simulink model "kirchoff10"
settings: Solver=ode23s  StartTime=0.0  StopTime=1  RelTol=1e-3
libraries: fl_lib x14, nesl_utility x7, powerlib x1

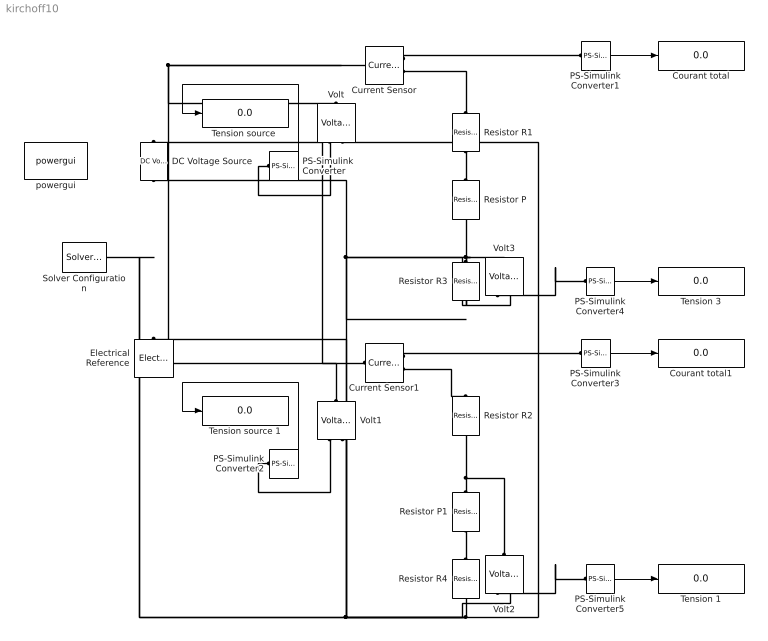
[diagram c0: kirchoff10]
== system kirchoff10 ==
  Courant total : Display
  Courant total1 : Display
  Current Sensor : fl_lib/Electrical/Electrical Sensors/Current Sensor  i1_Log=off  v1_Log=off  LocalVarNames=|i1|v1  LocalVarDescs=|i1|v1  LocalVarLogging=[0 0]
  Current Sensor1 : fl_lib/Electrical/Electrical Sensors/Current Sensor  i1_Log=off  v1_Log=off  LocalVarNames=|i1|v1  LocalVarDescs=|i1|v1  LocalVarLogging=[0 0]
  DC Voltage Source : fl_lib/Electrical/Electrical Sources/DC Voltage Source  v0=10 V  i_Log=off  v_Log=off  LocalVarNames=|i|v  LocalVarDescs=|i|v  LocalVarLogging=[0 0]
  Electrical Reference : fl_lib/Electrical/Electrical Elements/Electrical Reference  i_Log=off  LocalVarNames=|i  LocalVarDescs=|i  LocalVarLogging=0
  PS-Simulink Converter{,2,4..5} (4 alike) : nesl_utility/PS-Simulink Converter  PhysicalDomain=network_engine_domain  LeftPortType=input  RightPortType=output  SubClassName=ps_output  Unit=V  AffineConversion=off
  PS-Simulink Converter1 : nesl_utility/PS-Simulink Converter  PhysicalDomain=network_engine_domain  LeftPortType=input  RightPortType=output  SubClassName=ps_output  Unit=A  AffineConversion=off
  PS-Simulink Converter3 : nesl_utility/PS-Simulink Converter  PhysicalDomain=network_engine_domain  LeftPortType=input  RightPortType=output  SubClassName=ps_output  Unit=A  AffineConversion=off
  Resistor P : fl_lib/Electrical/Electrical Elements/Resistor  R=10 kOhm  i_Log=off  v_Log=off  LocalVarNames=|i|v  LocalVarDescs=|i|v  LocalVarLogging=[0 0]
  Resistor P1 : fl_lib/Electrical/Electrical Elements/Resistor  R=10 kOhm  i_Log=off  v_Log=off  LocalVarNames=|i|v  LocalVarDescs=|i|v  LocalVarLogging=[0 0]
  Resistor R{1..4} (4 alike) : fl_lib/Electrical/Electrical Elements/Resistor  R=100 Ohm  i_Log=off  v_Log=off  LocalVarNames=|i|v  LocalVarDescs=|i|v  LocalVarLogging=[0 0]
  Solver Configuration : nesl_utility/Solver Configuration  PhysicalDomain=network_engine_domain  LeftPortType=input  RightPortType=generic  SubClassName=solver  UseCustomDae=off  DoDC=off  ResidualTolerance=1e-9  UseLocalSolver=off  LocalSolverChoice=NE_BACKWARD_EULER_ADVANCER  LocalSolverSampleTime=.001  DoFixedCost=off  MaxNonlinIter=3  MaxModeIter=2  LinearAlgebra=Sparse  Accelerate=off  Profile=off  UseLocalSampling=off  DelaysMemoryBudget=1024
  Tension 1 : Display
  Tension 3 : Display
  "Tension source " : Display
  Tension source 1 : Display
  Volt{,1..3} (4 alike) : fl_lib/Electrical/Electrical Sensors/Voltage Sensor  i1_Log=off  v1_Log=off  LocalVarNames=|i1|v1  LocalVarDescs=|i1|v1  LocalVarLogging=[0 0]
  powergui : powerlib/powergui  Priority=1  SimulationMode=Continuous  SolverType=Tustin  SampleTime=50e-6  frequency=60  SPID=off  DisableSnubberDevices=off  DisableRonSwitches=off  DisableVfSwitches=off  SwTol=0  Interpol=off  DisplayEquations=off  FunctionMessages=off  frequencyindice=17  Pbase=100e6  ErrMax=1e-4  Iterations=50  UnitsV=V  UnitsW=W  echomessages=off  HookPort=off  EnableUseOfTLC=off  x0status=blocks  RestoreLinks=warning  ResistiveCurrentMeasurement=off  Ylog=off  Xlog=on  ShowGrid=off  save=off  variable=ZData  ZoomFFT=off  StartTime=0.0  cycles=1  DisplayStyle=1  FreqAxis=off  MaxFrequency=1000  frequencyindicesteady=1  display=off  methode=off
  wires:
  PS-Simulink Converter1/1 -> Courant total/1
  PS-Simulink Converter/1 -> "Tension source "/1
  PS-Simulink Converter4/1 -> Tension 3/1
  PS-Simulink Converter3/1 -> Courant total1/1
  PS-Simulink Converter2/1 -> Tension source 1/1
  PS-Simulink Converter5/1 -> Tension 1/1
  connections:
  Volt/LConn1 -- Current Sensor/LConn1 -- DC Voltage Source/LConn1 -- Current Sensor1/LConn1 -- Volt1/LConn1
  Current Sensor/RConn1 -- PS-Simulink Converter1/LConn1
  Resistor R1/LConn1 -- Current Sensor/RConn2
  Volt/RConn1 -- PS-Simulink Converter/LConn1
  Volt3/RConn1 -- PS-Simulink Converter4/LConn1
  Resistor R3/LConn1 -- Volt3/LConn1 -- Resistor P/RConn1
  Resistor R1/RConn1 -- Resistor P/LConn1
  Resistor R4/RConn1 -- Volt2/RConn2 -- Volt1/RConn2 -- Volt3/RConn2 -- Resistor R3/RConn1 -- Volt/RConn2 -- Solver Configuration/RConn1 -- DC Voltage Source/RConn1 -- Electrical Reference/LConn1
  Resistor P1/RConn1 -- Resistor R4/LConn1
  Current Sensor1/RConn2 -- Resistor R2/LConn1
  Volt2/RConn1 -- PS-Simulink Converter5/LConn1
  Volt1/RConn1 -- PS-Simulink Converter2/LConn1
  Current Sensor1/RConn1 -- PS-Simulink Converter3/LConn1
  Resistor P1/LConn1 -- Volt2/LConn1 -- Resistor R2/RConn1
